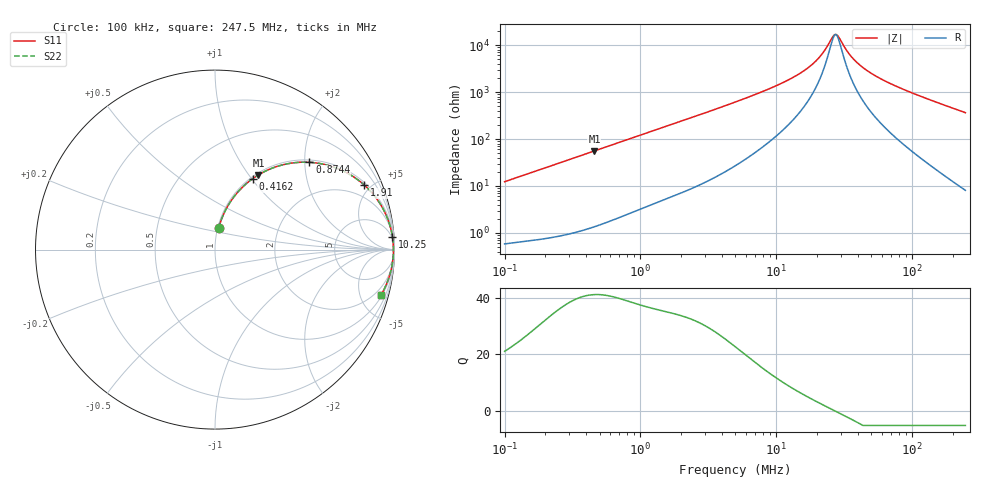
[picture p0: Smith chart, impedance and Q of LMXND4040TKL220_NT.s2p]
! LMXND4040TKL220_NT  S-PARAMETER MODEL  ( Standard Model )
! Model Generated by TAIYO YUDEN Corporation (https://www.yuden.co.jp/en/)
! Version 1.0
! TAIYO YUDEN Control No. 20250409
! Copyright(c) 2025 TAIYO YUDEN CO.,LTD. All Rights Reserved.
! Product Description (link to TY-COMPAS)
! https://ds.yuden.co.jp/TYCOMPAS/or/detail?pn=LMXND4040TKL220MNT&u=M
! Products Name : Inductors
! Characteristics :
!  Inductance : 22 [uH] , SRF(min) : 15 [MHz] , DC Resistance(max) : 0.348 [Ohm]
!  Rated Current : Saturation  900 [mA] , Temp Rise  1060 [mA] (40 [degC])
!  Case Size : 4.0 x 4.0 / 0.157 x 0.157 [mm/inch] , Thickness : 1.8 / 0.071 [mm/inch]
!  (Conditions: Temperature = 25 [degC] , DC Bias Current = 0 [A])
! External Node Assignments :
!  1  o---GGG---o  2
! GND o---------o GND
! Frequency Range : 0.1MHz  -  247.502633MHz  [ 402 STEP ]
# MHz S RI R 50
! Freq[MHz].  S11 Real  S11 Imag  S21 Real  S21 Imag  S12 Real  S12 Imag  S22 Real  S22 Imag
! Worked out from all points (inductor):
!   401 points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, 100 kHz to 247.5 MHz, reference 50 ohm
!   read as one part in series: L = 19.5 uH near 104 kHz
!   highest Q = 41.1 at 458.9 kHz (marker M1), where L = 19.3 uH
!   self-resonance near 27.22 MHz
!   S11 on the Smith chart (normalised r, x): 100 kHz: 1.01, +0.25; 416.2 kHz: 1.02, +1.01; 874.4 kHz: 1.06, +2.11; 1.91 MHz: 1.13, +4.57; 10.25 MHz: 3, +28; 247.5 MHz: 1.16, -7.26
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0.1  0.0205 0.12  0.9795 -0.12  0.9795 -0.12  0.0205 0.12
0.214227  0.0703 0.2411  0.9297 -0.2411  0.9297 -0.2411  0.0703 0.2411
0.37019  0.1746 0.3674  0.8254 -0.3674  0.8254 -0.3674  0.1746 0.3674
0.416225  0.2094 0.3948  0.7906 -0.3948  0.7906 -0.3948  0.2094 0.3948
0.458932  0.2423 0.4165  0.7577 -0.4165  0.7577 -0.4165  0.2423 0.4165
0.874417  0.5261 0.4864  0.4739 -0.4864  0.4739 -0.4864  0.5261 0.4864
1.370406  0.7246 0.4329  0.2754 -0.4329  0.2754 -0.4329  0.7246 0.4329
1.910189  0.8324 0.3591  0.1676 -0.3591  0.1676 -0.3591  0.8324 0.3591
4.974964  0.9672 0.1576  0.0328 -0.1576  0.0328 -0.1576  0.9672 0.1576
10.24934  0.9889 0.0697  0.0111 -0.0697  0.0111 -0.0697  0.9889 0.0697
14.28641  0.9922 0.0425  0.00785 -0.0425  0.00785 -0.0425  0.9922 0.0425
18.41681  0.9934 0.0249  0.00658 -0.0249  0.00658 -0.0249  0.9934 0.0249
21.95685  0.9939 0.0136  0.00612 -0.0136  0.00612 -0.0136  0.9939 0.0136
26.17735  0.9941 0.00281  0.00592 -0.00281  0.00592 -0.00281  0.9941 0.00281
27.75732  0.9941 -0.000766  0.00591 0.000766  0.00591 0.000766  0.9941 -0.000766
28.86326  0.9941 -0.00315  0.00591 0.00315  0.00591 0.00315  0.9941 -0.00315
34.41129  0.9939 -0.014  0.00609 0.014  0.00609 0.014  0.9939 -0.014
40.23208  0.9935 -0.024  0.00647 0.024  0.00647 0.024  0.9935 -0.024
50.86042  0.9925 -0.0401  0.0075 0.0401  0.0075 0.0401  0.9925 -0.0401
68.1772  0.9901 -0.0633  0.00993 0.0633  0.00993 0.0633  0.9901 -0.0633
120.1361  0.9782 -0.1246  0.0218 0.1246  0.0218 0.1246  0.9782 -0.1246
247.5026  0.9247 -0.2529  0.0753 0.2529  0.0753 0.2529  0.9247 -0.2529
